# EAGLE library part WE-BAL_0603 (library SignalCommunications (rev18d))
WE-BAL Multilayer Chip Balun Characteristics Low loss SMD Balun with balanced impedance of 50 to 200 Ω Operating temperature: –40 °C to +85 °C Power Capacity: 2 W max. Applications RF applications Wireless communication systems like Home RF, DECT, WLAN, Bluetooth, ZigBee … Details see: http://katalog.we-online.de/en/pbs/WE-BAL Updated by Dan Xu 2014-06-19 2014 (C) Wurth Elektronik
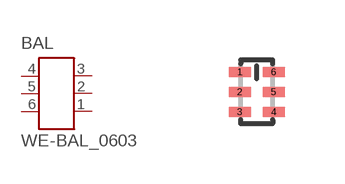
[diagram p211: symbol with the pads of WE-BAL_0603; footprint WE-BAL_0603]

Designator prefix BAL

## WE-BAL_0603_748411245, WE-BAL_0603_748412245, WE-BAL_0603_748415245  [WE-BAL_0603]
1  1  pas
2  2  pas
3  3  pas
4  4  pas
5  5  pas
6  6  pas

## Footprint WE-BAL_0603 (pad centres in mm)
Multilayer Chip Baluns WE-BAL
smd 0.55 x 0.25: 1 -0.425,0.5; 2 -0.425,0; 3 -0.425,-0.5; 4 0.425,-0.5; 5 0.425,0; 6 0.425,0.5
